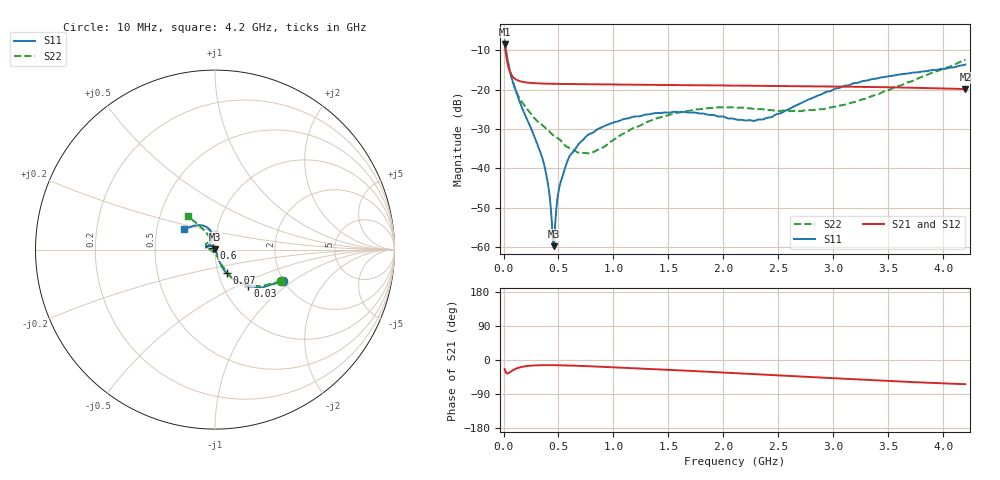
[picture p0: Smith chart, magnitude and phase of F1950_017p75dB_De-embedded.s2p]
! Integrated Device Technology
! Corporate Headquarters
! 6024 Silver Creek Valley Road
! San Jose, CA 95138  USA
! Phone:  1-408-284-8200
! Toll Free:  1-800-223-1366
! Webpage:  http://www.idt.com/
! Timing and RF Division
! 515 Groton Road, Suite 102
! Westford, MA 01886-6024
! Device:  F1950
! Description: 7-bit 0.25 dB Digital Step Attenuator
! Frequency:  150.0 -  4000.00 MHz
! Package:  4x4 mm Thin QFN Plastic Package: 24 pin
! Ports:  2 RF, 12 DC
!  Pin  1  = D0
!  Pin  2  = VDD
!  Pin  3  = Vmode
!  Pin  4  = GND
!  Pin  5  = RF1  =  Port 1
!  Pin  6  = GND
!  Pin  7  = GND
!  Pin  8  = GND
!  Pin  9  = GND
!  Pin 10  = GND
!  Pin 11  = GND
!  Pin 12  = GND
!  Pin 13  = GND
!  Pin 14  = RF2  =  Port 2
!  Pin 15  = GND
!  Pin 16  = LE
!  Pin 17  = CLK
!  Pin 18  = DATE
!  Pin 19  = D6
!  Pin 20  = D5
!  Pin 21  = D4
!  Pin 22  = D3
!  Pin 23  = D2
!  Pin 24  = D1
! State:  71
! Atten State:  17.75 dB
! Voltage:  +5.00 Volts
! Current:  Not Measured mA
! Data:  The device was measured on a the F195X evaluation board which has
!  individual transmission lines to the RF pins.  Data was collected
!  using a calibrated network analyzer.  The evaluation board was
!  de-embedded using a TRL calibration technique.
!  The reference plane is the edge of the package pin.
! Misc:  Board 2019
!  Action Tracker AT0250
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# GHz S dB R 50
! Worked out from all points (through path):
!   420 points, 10 MHz to 4.2 GHz, reference 50 ohm
!   highest |S21| = -8.45 dB at 10 MHz (marker M1); lowest = -19.9 dB at 4.2 GHz (marker M2)
!   group delay of S21, straight-line fit = 35.3 ps
!   lowest |S11| = -59.7 dB at 460 MHz (marker M3), VSWR 1.00, Z = 50 + j0.0913 ohm
!   |S11| at or under -10 dB: 22.75 MHz to end of sweep
!   |S22| runs from -36.2 to -7.8 dB; largest |S21 - S12| = 0.00018
!   S11 on the Smith chart (normalised r, x): 10 MHz: 1.99, -0.84; 30 MHz: 1.30, -0.57; 70 MHz: 1.10, -0.29; 600 MHz: 0.98, +0.02; 4.2 GHz: 0.69, +0.17
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0.01  -7.56 -24.7  -8.45 -23.7  -8.45 -23.7  -7.80 -25.7
0.03  -11.31 -48.0  -12.41 -35.3  -12.41 -35.3  -11.45 -47.6
0.07  -16.67 -63.7  -16.16 -29.8  -16.16 -29.8  -16.51 -62.1
0.16  -24.07 -69.3  -17.97 -18.6  -17.97 -18.6  -22.84 -68.8
0.36  -38.10 -58.2  -18.49 -13.6  -18.49 -13.6  -29.19 -74.0
0.41  -44.99 -54.3  -18.53 -13.6  -18.53 -13.6  -30.47 -74.6
0.44  -53.82 -38.4  -18.55 -13.6  -18.55 -13.6  -31.30 -77.3
0.46  -59.71 61.9  -18.56 -13.7  -18.56 -13.7  -31.75 -80.0
0.47  -54.09 91.8  -18.56 -13.7  -18.56 -13.8  -31.94 -81.2
0.49  -47.67 109.4  -18.57 -13.8  -18.57 -13.8  -32.27 -83.1
0.51  -44.46 117.4  -18.58 -14.0  -18.58 -14.0  -32.66 -84.1
0.6  -36.94 126.6  -18.62 -14.6  -18.62 -14.6  -34.82 -97.4
0.71  -33.08 131.9  -18.66 -15.7  -18.66 -15.7  -36.06 -118.0
0.81  -30.97 136.4  -18.69 -16.8  -18.69 -16.8  -35.94 -141.6
0.99  -28.46 144.2  -18.74 -19.1  -18.74 -19.1  -33.00 -171.1
1.41  -25.97 161.2  -18.85 -24.7  -18.85 -24.7  -27.16 164.7
1.74  -25.85 167.2  -18.92 -29.3  -18.92 -29.3  -25.07 155.8
2.11  -27.57 155.6  -19.00 -34.8  -19.00 -34.8  -24.60 146.2
2.43  -27.05 122.5  -19.08 -39.4  -19.08 -39.4  -25.22 135.9
2.81  -22.14 102.6  -19.18 -45.2  -19.17 -45.2  -25.23 120.3
3.51  -16.59 115.9  -19.42 -55.5  -19.42 -55.5  -20.08 116.6
4.2  -13.69 145.5  -19.90 -63.8  -19.89 -63.9  -12.45 129.0
